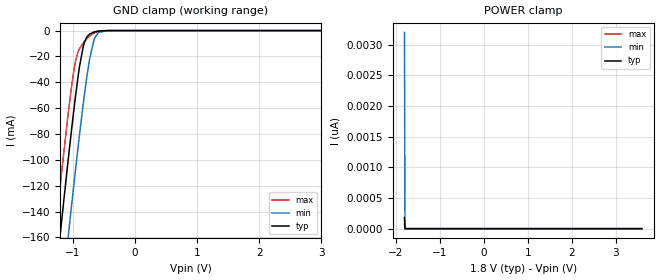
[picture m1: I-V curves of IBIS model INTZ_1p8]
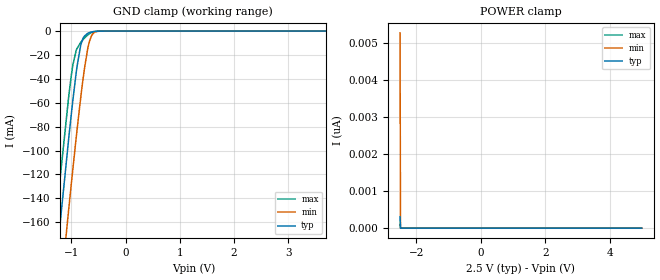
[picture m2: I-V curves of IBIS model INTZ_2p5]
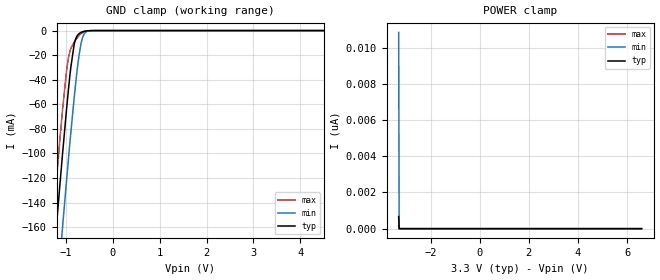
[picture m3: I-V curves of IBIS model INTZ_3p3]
|Texas Instruments Incorporated
| Low Voltage 4-channel I2C and SMbus Switch With Interrupt Logic and Reset
| Functions
| part#   Digital Voltage Range   Package-type   #pins
| TCA9544APWR   1.65V - 5.5V   TSSOP   20
[IBIS Ver]   4.1
[File name]   tca9544a.ibs
[File Rev]   1.0
[Date]   04/09/2014
[Source]
| Texas Instruments Incorporated.
| 12500 TI Blvd
| Dallas, TX -75243
[Notes]   Revision History:
| Rev 1.0: 04/09/2014
| - Initial version of the model
| - Model generated from simulations in TISPICE
| - C_comp although listed in numerical order of value are
|   obtained from varying PVT conditions. For PVT conditions for
|   each specific value refer the buffer description under
|   respective [Model]. IBIS model user is responsible for using
|   appropriate C_comp to simulate for Signal Integrity.
| - Warnings regarding combined/Non-monotonicity of various models have been
|   reviewd and considered minor and can be ignored.
| - Model names with a trailing _1p8 contains the model for 1.8V operation.
|   Model names with a trailing _2p5 contains the model for 2.5V operation.
|   Model names with a trailing _3p3 contains the model for 3.3V operation.
|   Model names with a trailing _5p0 contains the model for 5.0V operation.
[Disclaimer]
| This model is designed as an aid for customers of Texas Instruments.
| TI and its licensors and suppliers make no warranties, either expressed
| or implied, with respect to this  model, including the warranties of
| merchantability or fitness for a particular purpose. The model is
| provided solely on an "as is" basis. The entire risk as to its quality
| and performance is with the customer.
[Copyright]
 (C) Copyright 2014 Texas Instruments Incorporated.All rights reserved.
|   Device
[Component]   TCA9544A
[Manufacturer]   TI
[Package]
|   typ   min   max
R_pkg   0.2760   0.2481   0.3046
L_pkg   3.3282nH   2.7997nH   3.9247nH
C_pkg   0.5177pF   0.4340pF   0.6204pF
[Pin]  signal_name   model_name   R_pin   L_pin   C_pin
1   A0   INTZ   0.27705   3.9239nH   0.62039pF
2   A1   INTZ   0.29069   3.61994nH   0.58902pF
3   A2   INTZ   0.30336   3.38742nH   0.49574pF
4   INT0   INTZ   0.26732   2.93561nH   0.45031pF
5   SD0   NC   0.24822   2.80047nH   0.43402pF
6   SC0   NC   0.24835   2.80223nH   0.43419pF
7   INT1   INTZ   0.26776   2.94167nH   0.45066pF
8   SD1   NC   0.30412   3.40132nH   0.4969pF
9   SC1   NC   0.28062   3.56472nH   0.58792pF
10   GND   GND   0.27345   3.90184nH   0.61458pF
11   INT2   INTZ   0.27644   3.92467nH   0.61769pF
12   SD2   NC   0.28168   3.57073nH   0.59079pF
13   SC2   NC   0.3046   3.40163nH   0.49809pF
14   INT3   INTZ   0.2681   2.94434nH   0.45076pF
15   SD3   NC   0.24848   2.80338nH   0.43416pF
16   SC3   NC   0.24811   2.79969nH   0.43398pF
17   INTB   INTZ_OP   0.267   2.93308nH   0.4502pF
18   SCL   SCL   0.30288   3.38722nH   0.49465pF
19   SDA   SDA   0.28576   3.59983nH   0.59065pF
20   VCC   POWR   0.27654   3.92033nH   0.61847pF
|   Model Selectors
[Model Selector]  SDA
SDA_5p0   SDA buffer at 5.0V operation
SDA_3p3   SDA buffer at 3.3V operation
SDA_2p5   SDA buffer at 2.5V operation
SDA_1p8   SDA buffer at 1.8V operation
[Model Selector]  SCL
SCL_5p0   SCL buffer at 5.0V operation
SCL_3p3   SCL buffer at 3.3V operation
SCL_2p5   SCL buffer at 2.5V operation
SCL_1p8   SCL buffer at 1.8V operation
[Model Selector]  INTZ_OP
INTZ_OP_5p0   INTZ_OP buffer at 5.0V operation
INTZ_OP_3p3   INTZ_OP buffer at 3.3V operation
INTZ_OP_2p5   INTZ_OP buffer at 2.5V operation
INTZ_OP_1p8   INTZ_OP buffer at 1.8V operation
[Model Selector]  INTZ
INTZ_5p0   Input buffer at 5.0V operation
INTZ_3p3   Input buffer at 3.3V operation
INTZ_2p5   Input buffer at 2.5V operation
INTZ_1p8   Input buffer at 1.8V operation
| Models and submodels in the file (16): INTZ_1p8 (Input), INTZ_2p5 (Input), INTZ_3p3 (Input), INTZ_5p0 (Input), INTZ_OP_1p8 (Open_drain), INTZ_OP_2p5 (Open_drain), INTZ_OP_3p3 (Open_drain), INTZ_OP_5p0 (Open_drain), SCL_1p8 (Input), SCL_2p5 (Input), SCL_3p3 (Input), SCL_5p0 (Input), SDA_1p8 (I/O_open_drain), SDA_2p5 (I/O_open_drain), SDA_3p3 (I/O_open_drain), SDA_5p0 (I/O_open_drain)
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|   Model
[Model]   INTZ_1p8
Model_type   Input
Vinl = 0.54
Vinh = 1.26
|   typ   min   max
C_comp   1.378pF   1.292pF   1.466pF
[Voltage Range]   1.8   1.65   1.95
[Temperature Range]   27   125   -40
[Power Clamp Reference]   1.8   1.65   1.95
[GND Clamp Reference]   -0   -0   -0
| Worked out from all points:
|   GND clamp passes 1 mA (typ) near -0.65 V on its own axis
[GND Clamp]
|   Voltage   I(typ)   I(min)   I(max)
-1.8V     -444.5mA   -504.4mA   -407.1mA
-1.438V   -270.2mA   -330.8mA   -232.3mA
-1.222V   -168.5mA   -229.1mA   -130.8mA
-1.184V   -151.1mA   -211.6mA   -113.6mA
-1.071V   -100.1mA   -159.8mA   -64.28mA
-968.4mV  -56.83mA   -114.3mA   -27.68mA
-887.4mV  -27.43mA   -79.99mA   -13.89mA
-811.8mV  -9.407mA   -50.31mA   -8.666mA
-725.4mV  -2.729mA   -21.86mA   -4.347mA
-644.4mV  -935.9uA   -5.718mA   -1.642mA
-450mV    -25.03uA   -60uA      -30.72uA
3.595V    0A         0A         0A
[POWER Clamp]
|   Voltage   I(typ)   I(min)   I(max)
-1.8V     179.4pA    3.2nA      72.27pA
-1.789V   0A         0A         0A
-1.784V   0A         0A         0A
3.595V    0A         0A         0A
|   Model
[Model]   INTZ_2p5
Model_type   Input
Vinl = 0.75
Vinh = 1.75
|   typ   min   max
C_comp   1.378pF   1.292pF   1.466pF
[Voltage Range]   2.5   2.3   2.7
[Temperature Range]   27   125   -40
[Power Clamp Reference]   2.5   2.3   2.7
[GND Clamp Reference]   -0   -0   -0
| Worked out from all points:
|   GND clamp passes 1 mA (typ) near -0.65 V on its own axis
[GND Clamp]
|   Voltage   I(typ)   I(min)   I(max)
-2.5V     -787mA     -845.5mA   -750.7mA
-1.48V    -290.1mA   -350.6mA   -252.3mA
-1.285V   -197.8mA   -258.4mA   -159.9mA
-1.218V   -166.4mA   -226.9mA   -128.7mA
-1.052V   -92.02mA   -151.4mA   -56.8mA
-970mV    -57.47mA   -115mA     -28.12mA
-910mV    -34.93mA   -89.36mA   -16.29mA
-827.5mV  -12.06mA   -56.22mA   -9.593mA
-692.5mV  -1.8mA     -13.74mA   -3.073mA
-610mV    -552.2uA   -2.69mA    -947uA
-475mV    -43.19uA   -107.4uA   -55.89uA
4.992V    0A         0A         0A
[POWER Clamp]
|   Voltage   I(typ)   I(min)   I(max)
-2.5V     306.4pA    5.259nA    105.1pA
-2.485V   0A         0A         0A
-2.478V   0A         0A         0A
4.992V    0A         0A         0A
|   Model
[Model]   INTZ_3p3
Model_type   Input
Vinl = 0.99
Vinh = 2.31
|   typ   min   max
C_comp   1.378pF   1.292pF   1.466pF
[Voltage Range]   3.3   3   3.6
[Temperature Range]   27   125   -40
[Power Clamp Reference]   3.3   3   3.6
[GND Clamp Reference]   -0   -0   -0
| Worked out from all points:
|   GND clamp passes 1 mA (typ) near -0.65 V on its own axis
[GND Clamp]
|   Voltage   I(typ)   I(min)   I(max)
-3.3V     -1.182A    -1.239A    -1.146A
-1.34V    -223.5mA   -284.2mA   -185.6mA
-1.28V    -195.6mA   -256.3mA   -157.7mA
-1.211V   -163.4mA   -223.9mA   -125.7mA
-1.082V   -105.1mA   -164.9mA   -69mA
-943.8mV  -47.25mA   -103.7mA   -21.79mA
-825mV    -11.6mA    -55.27mA   -9.442mA
-735.9mV  -3.119mA   -24.84mA   -4.801mA
-656.7mV  -1.116mA   -7.317mA   -1.956mA
-577.5mV  -319uA     -1.25mA    -520.2uA
-409.2mV  -9.659uA   -23.55uA   -10.74uA
6.59V     0A         0A         0A
[POWER Clamp]
|   Voltage   I(typ)   I(min)   I(max)
-3.3V     664pA      10.84nA    162.7pA
-3.28V    0A         0A         0A
-3.27V    0A         0A         0A
6.59V     0A         0A         0A
